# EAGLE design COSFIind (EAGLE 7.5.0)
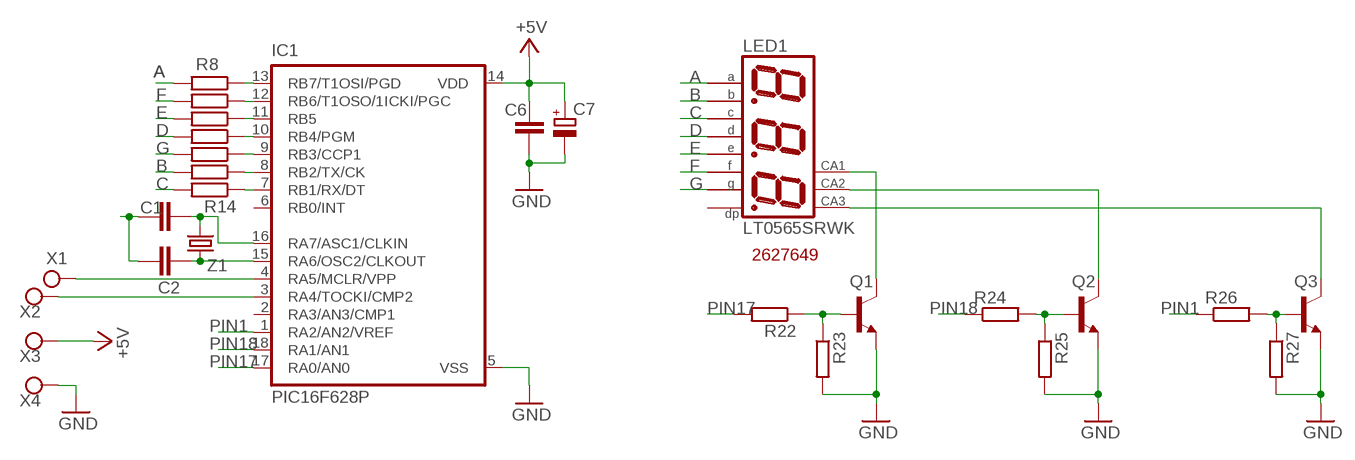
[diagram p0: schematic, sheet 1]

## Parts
C1  C-EUC1206  [C1206]
C2  C-EUC1206  [C1206]
C6  C-EUC1206  [C1206]
C7  CPOL-EUE2.5-7  [E2,5-7]
IC1  PIC16F628P  [DIL18]
LED1  LT0565SRWK  BA56-12EWA  [BX56-12]
Q1  BC337  [TO92]
Q2  BC337  [TO92]
Q3  BC337  [TO92]
R8  R-EU_0204/7  [0204/7]
R9  R-EU_0204/7  [0204/7]
R10  R-EU_0204/7  [0204/7]
R11  R-EU_0204/7  [0204/7]
R12  R-EU_0204/7  [0204/7]
R13  R-EU_0204/7  [0204/7]
R14  R-EU_0204/7  [0204/7]
R22  R-EU_0204/7  [0204/7]
R23  R-EU_0204/7  [0204/7]
R24  R-EU_0204/7  [0204/7]
R25  R-EU_0204/7  [0204/7]
R26  R-EU_0204/7  [0204/7]
R27  R-EU_0204/7  [0204/7]
X1  CONNWIRE  [CONNWIRE]
X2  CONNWIRE  [CONNWIRE]
X3  CONNWIRE  [CONNWIRE]
X4  CONNWIRE  [CONNWIRE]
Z1  CRYSTALHC49S  [HC49/S]

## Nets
+5V: C6.2 C7.+ IC1.14(VDD) X3.P$1
A: LED1.11(A) R8.2
B: LED1.7(B) R13.2
C: LED1.4(C) R14.2
D: LED1.2(D) R11.2
E: LED1.1(E) R10.2
F: LED1.10(F) R9.2
G: LED1.5(G) R12.2
GND: C1.2 C2.2 C6.1 C7.- IC1.5(VSS) Q1.1(E) Q2.1(E) Q3.1(E) R23.2 R25.2 R27.2 X4.P$1
N$1: LED1.12(CA) Q1.3(C)
N$2: LED1.9(CA) Q2.3(C)
N$3: LED1.8(CA) Q3.3(C)
N$4: C2.1 IC1.15(RA6/OSC2/CLKOUT) Z1.1
N$17: IC1.3(RA4/TOCKI/CMP2) X2.P$1
N$18: IC1.4(RA5/MCLR/VPP) X1.P$1
N$20: C1.1 IC1.16(RA7/ASC1/CLKIN) Z1.2
N$21: IC1.13(RB7/T1OSI/PGD) R8.1
N$22: Q1.2(B) R22.1 R23.1
N$23: IC1.12(RB6/T1OSO/1ICKI/PGC) R9.1
N$24: IC1.11(RB5) R10.1
N$25: IC1.10(RB4/PGM) R11.1
N$26: IC1.9(RB3/CCP1) R12.1
N$27: IC1.8(RB2/TX/CK) R13.1
N$28: IC1.7(RB1/RX/DT) R14.1
N$30: Q2.2(B) R24.2 R25.1
N$32: Q3.2(B) R26.2 R27.1
PIN1: IC1.1(RA2/AN2/VREF) R26.1
PIN17: IC1.17(RA0/AN0) R22.2
PIN18: IC1.18(RA1/AN1) R24.1
Unconnected: IC1.2(RA3/AN3/CMP1) IC1.6(RB0/INT) LED1.3(DP)

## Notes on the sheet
- 2627649

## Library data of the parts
C1 C2 C6 = rcl:C-EU: CAPACITOR, European symbol
C7 = rcl:CPOL-EU: POLARIZED CAPACITOR, European symbol
IC1 = microchip:PIC16*F62: FLASH-Based 8-Bit CMOS Microcontroller Source: http://ww1.microchip.com/downloads/en/DeviceDoc/40300C.pdf; MF: MICROCHIP; MPN: PIC16F628-20/P; OC_FARNELL: 9760423; OC_NEWARK: 23C4982
LED1 = display-kingbright:B?56-12*WA: 14.22mm (0.56INCH) THREE DIGIT NUMERIC DISPLAY Source: http://www.kingbright.com .. BA56-11EWA(Ver1189474895.pdf; OC_FARNELL: unknown; OC_NEWARK: unknown
Q1-Q3 = transistor:BC337: NPN TRANSISTOR
R8-R14 R22-R27 = rcl:R-EU_: RESISTOR, European symbol
X1-X4 = connholes:CONNWIRE
Z1 = crystal:CRYSTAL: CRYSTAL; OC_FARNELL: 1667008; OC_NEWARK: unknown

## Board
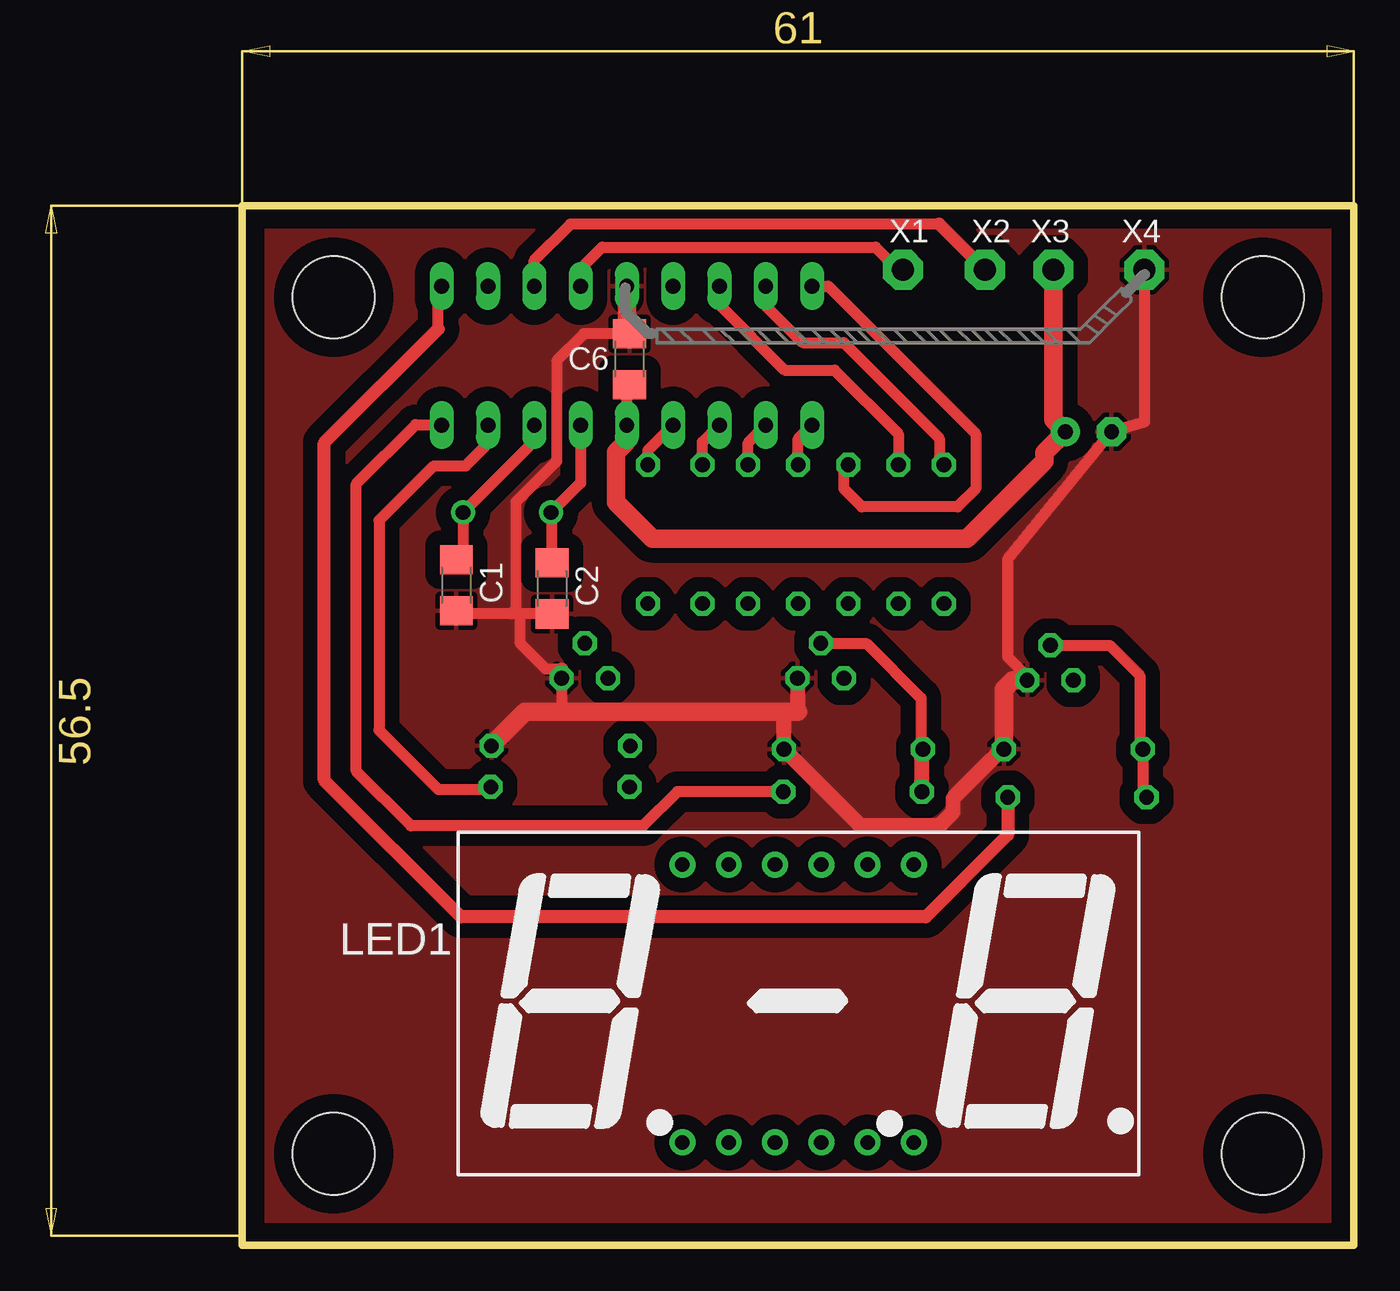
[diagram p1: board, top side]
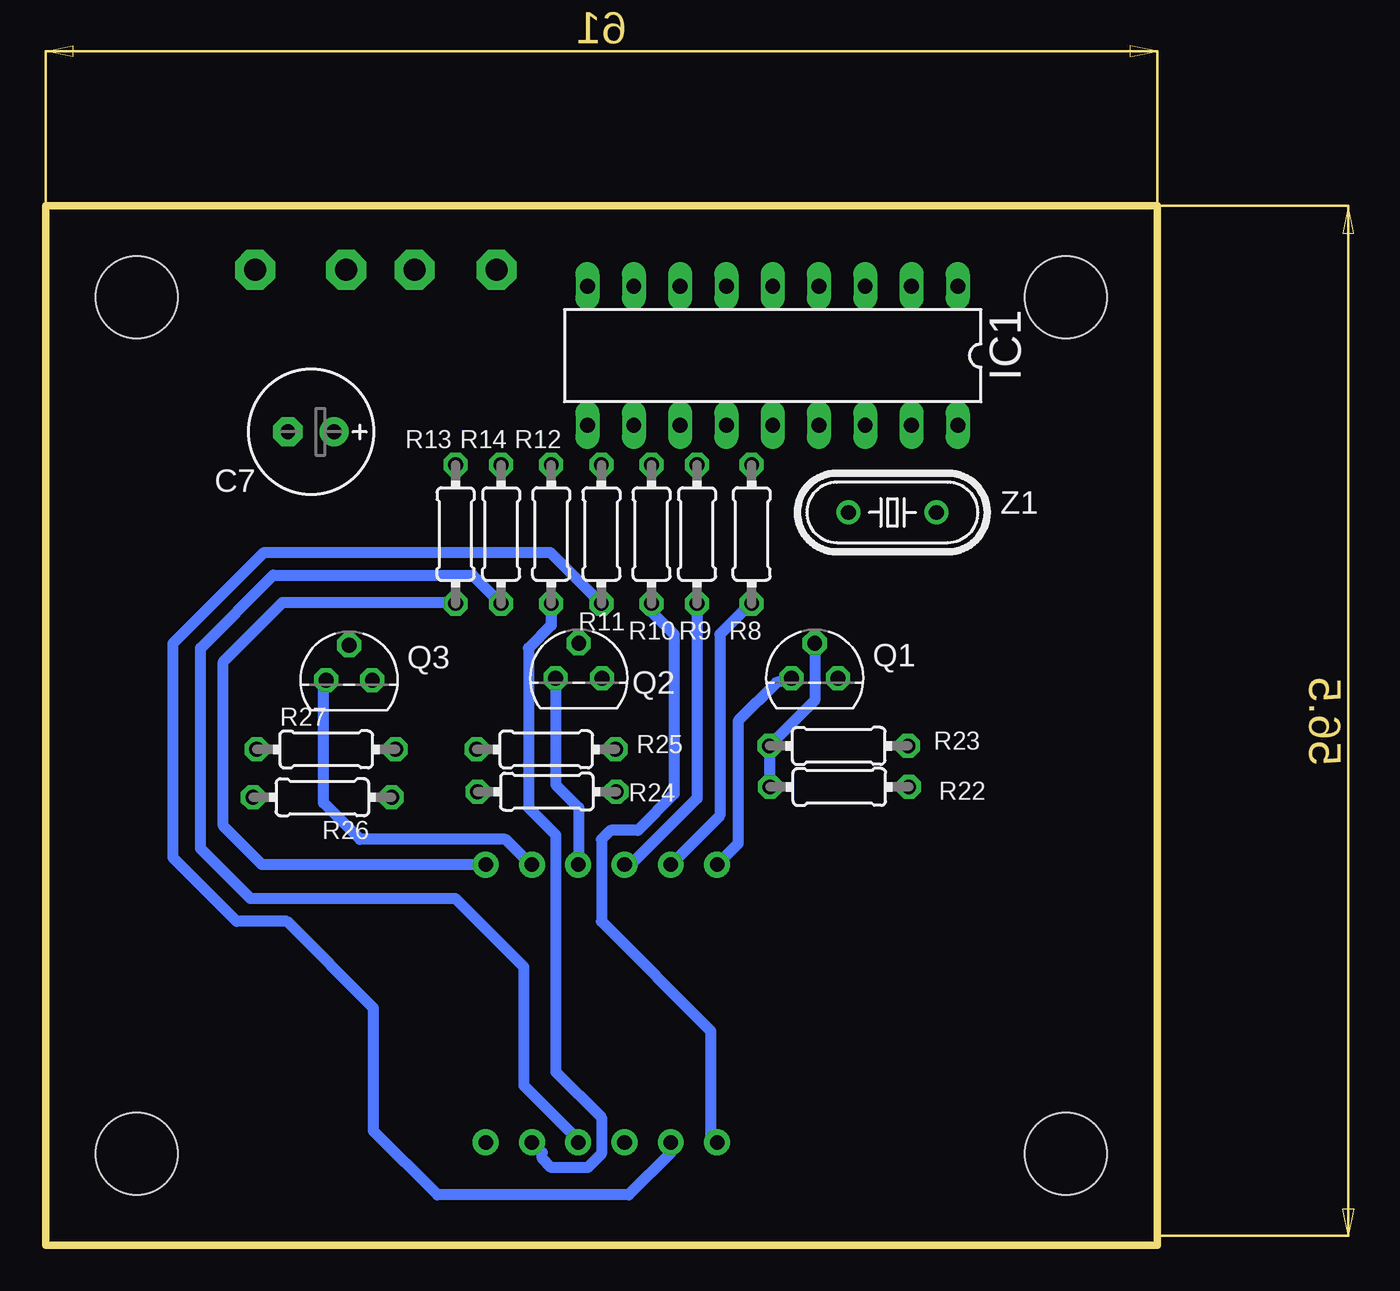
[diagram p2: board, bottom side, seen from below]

Size 71.8 x 65.8 mm. Coordinates in mm from the lower left corner, seen from the top.
Outline: 10.8,0 10.8,57 71.8,57 71.8,0 10.8,0
Copper layers (1*16): Top 0.035mm / dielectric 1.5mm / Bottom 0.035mm
Design rules "default": minimum track width 10mil, minimum drill 24mil, track to track 8mil, track to pad 8mil, pad to pad 8mil, via to via 8mil, smd to smd 8mil, copper to edge 40mil, drill to drill 8mil, minimum pad ring 10mil, minimum via ring 8mil, stop-mask expansion 4mil, vias tented up to drill 0mil, thermal gap 10mil
Holes 4.5 mm at 15.8,52 66.8,5 15.8,5 66.8,52

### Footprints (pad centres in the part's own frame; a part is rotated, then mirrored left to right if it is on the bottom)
C1206 = smd 1.6 x 1.8: 1 -1.4,0; 2 1.4,0
E2,5-7 = drill 0.813 pad 1.6: + -1.27,0 | drill 0.813 pad 1.6 octagon: - 1.27,0
DIL18 = drill 0.813 long: 1 -10.16,-3.81; 2 -7.62,-3.81; 3 -5.08,-3.81; 4 -2.54,-3.81; 5 0,-3.81; 6 2.54,-3.81; 7 5.08,-3.81; 8 7.62,-3.81; 9 10.16,-3.81; 10 10.16,3.81; 11 7.62,3.81; 12 5.08,3.81; 13 2.54,3.81; 14 0,3.81; 15 -2.54,3.81; 16 -5.08,3.81; 17 -7.62,3.81; 18 -10.16,3.81
BX56-12 = drill 0.8 pad 1.422: 1 -6.35,-7.62; 2 -3.81,-7.62; 3 -1.27,-7.62; 4 1.27,-7.62; 5 3.81,-7.62; 6 6.35,-7.62; 7 6.35,7.62; 8 3.81,7.62; 9 1.27,7.62; 10 -1.27,7.62; 11 -3.81,7.62; 12 -6.35,7.62
TO92 = drill 0.813 octagon: 1 1.27,0; 2 0,1.905; 3 -1.27,0
0204/7 = drill 0.813 octagon: 1 -3.81,0; 2 3.81,0
CONNWIRE = drill 1.2 pad 2.184 octagon: P$1 0,0
HC49/S = drill 0.813: 1 -2.413,0; 2 2.413,0

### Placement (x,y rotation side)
C1  22.54,36.19 270 top
C2  27.79,36.02 270 top
C6  32.04,48.6 270 top
C7  57.23,44.61 180 bottom
IC1  31.9,48.79 180 bottom
LED1  41.3,13.25 0 top
Q1  29.59,31.1 0 bottom
Q2  42.54,31.1 0 bottom
Q3  55.14,30.99 0 bottom
R8  33.05,39 270 bottom
R9  36.05,39 270 bottom
R10  38.55,39 270 bottom
R11  41.3,39 270 bottom
R12  44.05,39 270 bottom
R13  49.3,39 270 bottom
R14  46.8,39 270 bottom
R22  28.24,25.13 0 bottom
R23  28.28,27.38 0 bottom
R24  44.29,24.87 180 bottom
R25  44.33,27.19 0 bottom
R26  56.61,24.56 180 bottom
R27  56.4,27.19 0 bottom
X1  47.05,53.5 0 top
X2  51.55,53.5 0 top
X3  55.3,53.5 0 top
X4  60.3,53.5 0 top
Z1  25.33,40.19 0 bottom

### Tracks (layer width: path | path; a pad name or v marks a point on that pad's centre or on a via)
+5V
  Top 0.61: IC1.14 31.9,47.06 C6.2
  Top 1.016: IC1.14 31.9,44.1 31.3,43.5 31.3,40.75 33.3,38.75 50.55,38.75 54.8,43 54.8,43.45 C7.+ 55.3,45.27 X3.P$1
A
  Bottom 0.61: R8.2 33.11,35.19 34.8,33.5 34.8,23.56 LED1.11
B
  Bottom 0.61: LED1.7 59.92,20.87 62.05,23 62.05,32 58.8,35.25 49.36,35.25 R13.2
C
  Bottom 0.61: LED1.4 42.57,5.77 45.55,8.75 45.55,15.25 49.3,19 60.55,19 63.3,21.75 63.3,32.75 59.3,36.75 48.36,36.75 R14.2
D
  Bottom 0.61: LED1.2 37.49,5.06 39.8,2.75 50.3,2.75 53.8,6.25 53.8,13 58.55,17.75 61.3,17.75 64.8,21.25 64.8,33 59.8,38 44.11,38 R11.2
E
  Bottom 0.61: R10.2 38.55,34.75 37.3,33.5 37.3,24.75 39.3,22.75 40.8,22.75 41.3,22.25 41.3,17.75 35.3,11.75 35.3,5.98 LED1.1
F
  Bottom 0.61: R9.2 36.05,24.5 39.55,21 39.9,21 LED1.10
G
  Bottom 0.61: R12.2 44.05,34 45.3,32.75 45.3,24 43.8,22.5 43.8,9.5 41.3,7 41.3,5 42.05,4.25 44.05,4.25 44.55,4.75 44.55,5.07 LED1.5
GND
  Top 0.61: Q1.1 28.32,29.73 28.8,29.25 | C2.2 26.05,34.62 | 26.05,34.62 25.55,34.62 | 25.55,34.62 22.71,34.62 C1.2 | 28.32,31.59 27.46,31.59 26.05,33 26.05,34.62 | C6.1 29.55,50 28.05,48.5 28.05,43 25.8,40.75 25.8,34.87 25.55,34.62 | Q3.1 53.87,31.18 52.8,32.25 52.8,37.64 C7.- 60.3,45.14 X4.P$1
  Top 0.7: Q1.1 28.32,31.59
  Top 0.813: Q2.1 41.27,29.28 41.3,29.25 | 40.8,29.25 40.52,28.97 R25.2 44.71,23 49.05,23 49.8,23.75 49.8,24.5 52.49,27.19 R27.2
  Top 1.016: R23.2 24.46,27.41 26.3,29.25 28.8,29.25 40.8,29.25 41.3,29.25 | R27.2 52.59,30.5 53.08,30.99 Q3.1 | IC1.5 31.9,50.14 C6.1
  pour Top (isolate 0.813): 11.55,56.25 71.05,56.25 71.05,0.75 11.3,0.75 11.3,56.25
N$1
  Bottom 0.61: Q1.3 31.7,30.85 33.8,28.75 33.8,22.02 LED1.12
N$2
  Bottom 0.61: Q2.3 43.81,25.26 42.55,24 42.55,20.89 LED1.9
N$3
  Bottom 0.61: LED1.8 45.17,20.87 46.55,22.25 54.55,22.25 56.55,24.25 56.55,30.85 Q3.3
N$4
  Top 0.61: C2.1 27.79,40.14 Z1.1 29.36,41.81 IC1.15
N$17
  Top 0.61: 49.05,56 28.8,56 26.82,54.02 IC1.3
  Top 0.7: X2.P$1 49.05,56
N$18
  Top 0.61: X1.P$1 46.8,53.5 45.55,54.75 30.55,54.75 29.36,53.56 IC1.4 29.3,53.16
N$20
  Top 0.61: C1.1 22.92,37.97 Z1.2 26.82,44.09 IC1.16
N$21
  Top 0.61: R8.1 33.05,43.59 IC1.13
N$22
  Bottom 0.61: Q1.2 29.59,29.88 R23.1 32.09,25.16 R22.1
N$23
  Top 0.61: R9.1 36.05,44.05 IC1.12
N$24
  Top 0.61: R10.1 38.55,44.01 IC1.11
N$25
  Top 0.61: R11.1 41.3,44.22 IC1.10
N$26
  Top 0.61: R12.1 43.8,42.56 43.8,41.5 44.8,40.5 50.05,40.5 51.05,41.5 51.05,44.5 42.95,52.6 IC1.9
N$27
  Top 0.61: IC1.8 39.52,51.53 41.55,49.5 43.8,49.5 49.05,44.25 49.05,43.06 R13.1
N$28
  Top 0.61: IC1.7 36.98,51.57 40.55,48 43.3,48 46.8,44.5 R14.1
N$30
  Top 0.61: Q2.2 45.05,33.01 48.05,30 48.05,27.28 R25.1
  Top 0.813: R24.2 48.1,27.15 R25.1
  Bottom 0.813: 48.1,27.15 R25.1
N$32
  Top 0.61: R26.2 60.21,24.77 R27.1 60.05,27.35 60.05,31.25 58.41,32.9 Q3.2
PIN1
  Top 0.61: 21.55,50.25 21.55,52.41 IC1.1
  Top 0.7: R26.1 52.8,22.5 48.3,18 22.8,18 15.3,25.5 15.3,44 21.55,50.25
PIN17
  Top 0.61: R22.2 24.3,25 21.55,25 18.3,28.25 18.3,39.75 21.3,42.75 23.05,42.75 24.3,44 24.3,44.96 IC1.17
PIN18
  Top 0.61: R24.1 34.67,24.87 32.8,23 20.05,23 17.05,26 17.05,41.75 20.3,45 21.72,45 IC1.18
